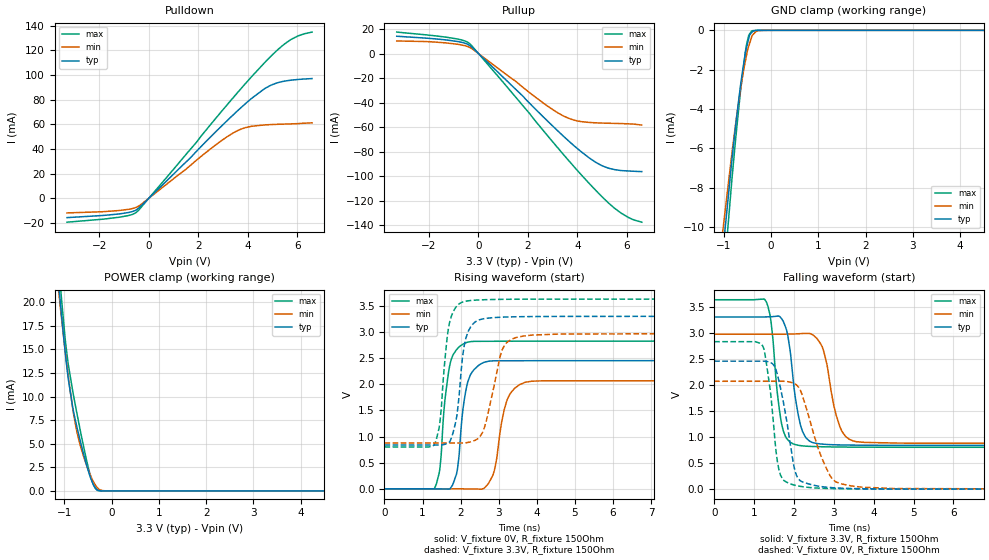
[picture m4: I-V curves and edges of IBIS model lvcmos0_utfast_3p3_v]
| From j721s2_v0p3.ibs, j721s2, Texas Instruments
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|   utfast_3p3_v
[Model]   lvcmos0_utfast_3p3_v
Model_type   I/O
Polarity   Non-Inverting
Enable   Active-High
Vinl = 0
Vinh = 0.8
Vmeas = 1.65
Vref = 3.3
Cref = 2pF
Rref = 100000
|   typ   min   max
C_comp   1.362pF   1.327pF   1.397pF
[Voltage Range]   3.3   2.97   3.63
[Temperature Range]   27   150   -40
[Pullup Reference]   3.3   2.97   3.63
[Pulldown Reference]   0   0   0
[Power Clamp Reference]   3.3   2.97   3.63
[GND Clamp Reference]   0   0   0
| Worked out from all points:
|   slope of the pulldown table from 0 to 0.495 V, typ, clamps not added: 51 ohm
|   slope of the pullup table from 0 to 0.495 V, typ, clamps not added: 51.8 ohm
|   GND clamp passes 1 mA (typ) near -0.53 V on its own axis
|   POWER clamp passes 1 mA (typ) near -0.41 V on its own axis
|   falling waveform, V_fixture 3.3V, R_fixture 150Ohm: 20-80 % time 261ps typ, 333ps min, 219ps max; typ from 3.3 V to 0.838 V
|   rising waveform, V_fixture 0V, R_fixture 150Ohm: 20-80 % time 224ps typ, 295ps min, 211ps max; typ from 0 V to 2.45 V
|   rising waveform, V_fixture 3.3V, R_fixture 150Ohm: 20-80 % time 230ps typ, 373ps min, 210ps max; typ from 0.838 V to 3.3 V
|   falling waveform, V_fixture 0V, R_fixture 150Ohm: 20-80 % time 331ps typ, 534ps min, 241ps max; typ from 2.45 V to 0 V
[Pulldown]
|   Voltage   I(typ)   I(min)   I(max)
-3.3V     -15.6mA    -11.79mA   -19.31mA
-1.191V   -12.61mA   -9.822mA   -15.27mA
-498.3mV  -9.27mA    -7.218mA   -11.32mA
1.67V     32.6mA     26.51mA    39.48mA
2.64V     52.68mA    42.35mA    63.27mA
3.61V     71.44mA    55.14mA    86.28mA
4.125V    80.57mA    58.37mA    98.01mA
4.67V     88.8mA     59.56mA    109.8mA
4.966V    92.01mA    59.9mA     115.9mA
5.758V    95.9mA     60.43mA    129mA
6.036V    96.46mA    60.66mA    131.8mA
6.6V      97.19mA    61.27mA    134.9mA
[GND Clamp]
|   Voltage   I(typ)   I(min)   I(max)
-3.3V     -92.62mA   -62.37mA   -137.3mA
-1.558V   -24.44mA   -21.27mA   -28.6mA
-825mV    -6.576mA   -6.239mA   -7.571mA
-726mV    -4.419mA   -4.397mA   -5.03mA
-646.8mV  -2.873mA   -3.062mA   -3.168mA
-537.9mV  -1.081mA   -1.53mA    -1.069mA
-468.6mV  -411.3uA   -800.1uA   -249.5uA
-448.8mV  -222.3uA   -649.5uA   -177.8uA
-399.3mV  -88.23uA   -272.9uA   -22.87uA
-310.2mV  -2.837uA   -44.94uA   -952.2nA
-132mV    -56.02nA   -1.517uA   -88.26nA
6.6V      0A         0A         0A
[Pullup]
|   Voltage   I(typ)   I(min)   I(max)
-3.3V     14.1mA     10.24mA    17.48mA
-1.34V    11.16mA    8.715mA    13.44mA
-686.4mV  9.185mA    7.036mA    11.1mA
-349.8mV  6.513mA    4.928mA    8.005mA
2.64V     -52.08mA   -40.67mA   -63.31mA
3.61V     -70.68mA   -52.55mA   -86.47mA
4.026V    -78.01mA   -55.09mA   -96.05mA
4.471V    -85.09mA   -56.22mA   -105.9mA
5.016V    -91.72mA   -56.75mA   -117.3mA
5.798V    -95.52mA   -57.16mA   -130.6mA
6.204V    -95.98mA   -57.52mA   -135.1mA
6.6V      -96.34mA   -58.35mA   -137.6mA
[POWER Clamp]
|   Voltage   I(typ)   I(min)   I(max)
-3.3V     165.9mA    145.4mA    188.3mA
-1.112V   21.57mA    20.89mA    23.69mA
-1.063V   18.87mA    18.55mA    20.64mA
-973.5mV  14.41mA    14.56mA    15.79mA
-914.1mV  11.87mA    12.11mA    13.39mA
-825mV    8.991mA    8.884mA    10.71mA
-735.9mV  6.868mA    6.368mA    8.325mA
-627mV    4.603mA    4.244mA    5.577mA
-468.6mV  1.77mA     1.94mA     2.021mA
-349.8mV  384.3uA    698.9uA    308.4uA
-290.4mV  90.1uA     296uA      37.22uA
6.6V      0A         0A         0A
[Ramp]
R_load = 150
|   typ   min   max
dV/dt_r   1.47177/2.23289e-10   1.24044/2.94604e-10   1.69589/2.1031e-10
dV/dt_f   1.4772/2.5801e-10   1.25557/3.29733e-10   1.69692/2.18347e-10
[Falling Waveform]
V_fixture = 3.3V
V_fixture_min = 2.97V
V_fixture_max = 3.63V
R_fixture = 150Ohm
C_fixture = 0F
|   Time   V(typ)   V(min)   V(max)
0s        3.3V       2.97V      3.63V
1.305ns   3.302V     2.97V      3.592V
1.425ns   3.305V     2.97V      3.205V
1.685ns   3.271V     2.97V      1.276V
1.99ns    2.027V     2.974V     865mV
2.31ns    978mV      2.985V     823.5mV
2.705ns   863.9mV    2.736V     813mV
3.145ns   848mV      1.212V     807.7mV
3.495ns   844.1mV    921.3mV    805.6mV
10ns      837.9mV    877.1mV    801.7mV
[Rising Waveform]
V_fixture = 0V
V_fixture_min = 0V
V_fixture_max = 0V
R_fixture = 150Ohm
C_fixture = 0F
|   Time   V(typ)   V(min)   V(max)
0s        97.29uV    253.8uV    50.59uV
1.315ns   65.81uV    229.6uV    9.788mV
1.45ns    -745.2uV   110.2uV    360.1mV
1.69ns    -4.524mV   124.7uV    2.264V
1.89ns    279.5mV    110.5uV    2.659V
2.155ns   1.946V     -1.287mV   2.799V
2.76ns    2.443V     140mV      2.822V
3.225ns   2.45V      1.707V     2.824V
3.69ns    2.451V     2.037V     2.825V
10ns      2.453V     2.068V     2.827V
[Rising Waveform]
V_fixture = 3.3V
V_fixture_min = 2.97V
V_fixture_max = 3.63V
R_fixture = 150Ohm
C_fixture = 0F
|   Time   V(typ)   V(min)   V(max)
0s        837.9mV    877.1mV    801.7mV
1.31ns    837.9mV    877mV      841.4mV
1.45ns    837.7mV    876.9mV    1.24V
1.645ns   869.5mV    876.9mV    2.886V
1.77ns    998.7mV    877mV      3.327V
2.045ns   2.487V     877.2mV    3.571V
2.58ns    3.25V      1.086V     3.616V
3.09ns    3.284V     2.655V     3.624V
3.455ns   3.291V     2.894V     3.627V
10ns      3.3V       2.97V      3.63V
[Falling Waveform]
|Gnd
V_fixture = 0V
V_fixture_min = 0V
V_fixture_max = 0V
R_fixture = 150Ohm
C_fixture = 0F
|   Time   V(typ)   V(min)   V(max)
0s        2.453V     2.068V     2.827V
1.215ns   2.453V     2.068V     2.745V
1.405ns   2.428V     2.068V     1.9V
1.615ns   2.101V     2.068V     404.1mV
1.92ns    808mV      2.048V     99mV
2.03ns    341.1mV    2.015V     73.91mV
2.155ns   163.9mV    1.903V     54.74mV
2.795ns   39.51mV    427.1mV    14.56mV
3.19ns    19.13mV    102.9mV    7.811mV
10ns      97.42uV    253.8uV    50.59uV
